// Automatisch erzeugter Code: NICHT EDITIEREN
FUNCTION CheckBounds : DINT
VAR_INPUT
	index, lower, upper: DINT;
END_VAR

// Automatisch erzeugter Code: Es handelt sich hierbei um einen Implementierungsvorschlag.
{noflow}
IF  index < lower THEN
	GVL_Check.nCntLower := GVL_Check.nCntLower + 1;
	CheckBounds := lower;
ELSIF  index > upper THEN
	GVL_Check.nCntUpper := GVL_Check.nCntUpper + 1;
	CheckBounds := upper;
ELSE  
	CheckBounds := index;
END_IF
{flow}

END_FUNCTION
